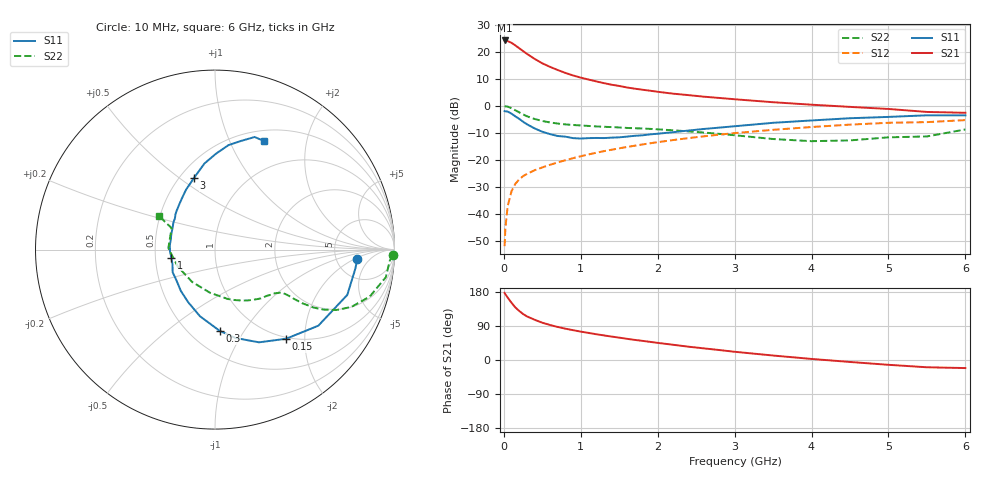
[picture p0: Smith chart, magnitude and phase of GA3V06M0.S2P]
! Infineon Technologies  Discrete & RF Semiconductors
! BF775
! Si NPN RF Bipolar Junction Transistor in SOT23
! VCE = 3 V  IC = 6 mA
! Common Emitter S-Parameters:  May  1996
# GHz  S  MA  R  50
!  f  S11  S21  S12  S22
! GHz  MAG  ANG  MAG  ANG  MAG  ANG  MAG  ANG
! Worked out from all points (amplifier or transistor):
!   36 points, 10 MHz to 6 GHz, reference 50 ohm
!   highest |S21| = 24.2 dB at 10 MHz (marker M1)
!   |S21| within 3 dB of that: start of sweep to 205.3 MHz
!   unconditionally stable (mu >= 1): 725.1 MHz to 3.484 GHz
!   at 250 MHz: K = 0.54, MSG = 23.2 dB, |S12| = -26.1 dB
!   at 1.4 GHz: K = 1.13, MAG = 9.9 dB, |S12| = -16.3 dB
!   at 6 GHz: K = 0.96, MSG = 1.4 dB, |S12| = -5.3 dB
!   S11 on the Smith chart (normalised r, x): 10 MHz: 8.01, -2.34; 150 MHz: 0.97, -1.62; 300 MHz: 0.69, -0.79; 1 GHz: 0.61, -0.06; 3 GHz: 0.59, +0.57; 6 GHz: 0.63, +1.35
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0.01  0.794 -3.9  16.22 177.0  0.0025 89.2  0.9899 -1.7
0.02  0.7892 -7.7  16.21 173.5  0.0054 85.2  0.9758 -3.7
0.05  0.7791 -18.9  15.78 164.7  0.0138 81.6  0.964 -9.2
0.1  0.7149 -36.4  14.66 151.0  0.0261 71.1  0.901 -16.9
0.15  0.6349 -51.5  13.12 138.6  0.0359 65.9  0.8242 -22.8
0.2  0.5719 -64.6  11.63 129.4  0.0433 62.1  0.7548 -26.5
0.25  0.5057 -76.9  10.3 121.3  0.0496 59.1  0.6916 -28.9
0.3  0.454 -86.6  9.162 115.1  0.0545 58.2  0.6394 -30.4
0.4  0.3807 -102.7  7.394 106.2  0.0638 57.0  0.5689 -31.6
0.5  0.3296 -116.8  6.113 98.4  0.072 57.0  0.5225 -31.9
0.6  0.2986 -129.6  5.262 92.4  0.0806 57.6  0.4904 -32.0
0.7  0.2751 -141.2  4.597 87.2  0.0889 58.2  0.4683 -32.2
0.8  0.2675 -151.9  4.059 82.7  0.0979 58.5  0.4514 -32.6
1  0.247 -169.7  3.32 74.9  0.1159 59.0  0.4313 -33.8
1.1  0.2511 -177.4  3.062 71.5  0.1252 59.1  0.4227 -35.0
1.6  0.2681 151.2  2.183 55.9  0.1724 57.4  0.3882 -41.4
2.2  0.3237 127.5  1.675 40.2  0.2313 52.9  0.351 -52.9
3  0.4171 106.2  1.32 21.7  0.3114 44.4  0.2843 -75.5
3.5  0.4833 97.0  1.163 11.8  0.3581 38.3  0.2419 -96.7
4.5  0.5872 82.6  0.953 -5.2  0.4471 25.3  0.228 -155.6
5.5  0.6651 70.6  0.768 -19.2  0.4976 10.4  0.27 153.6
6  0.6636 65.6  0.741 -21.3  0.5422 6.3  0.3639 149.1
